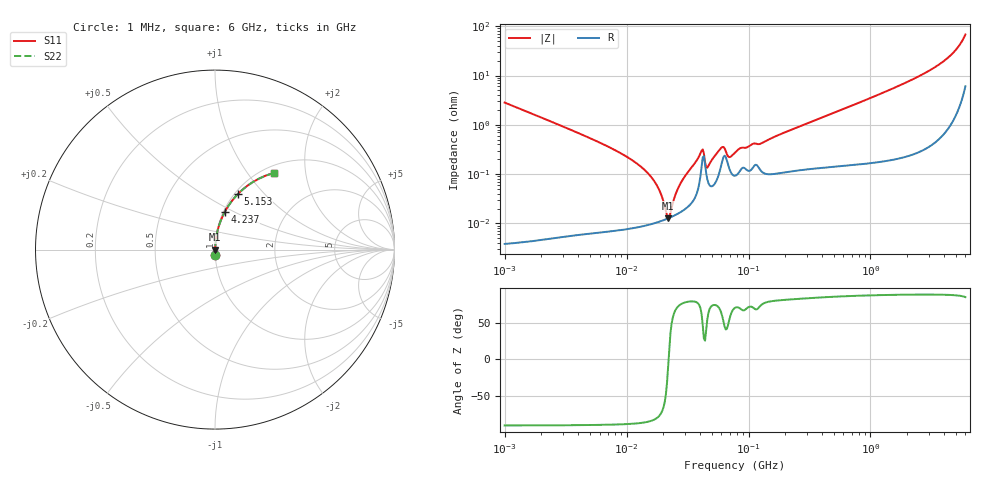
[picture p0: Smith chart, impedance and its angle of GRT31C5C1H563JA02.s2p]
!Murata Part Number: GRT31C5C1H563JA02
!These Parameters are Measured in Series Mode Connection
!Data Generated on Jun 19, 2026
!  o--ll--o
!Port1  Port2
!  o------o
!Operation Temp=25[degC], DC Bias Voltage=0[V]
!Freq. Start=1000[kHz] Stop=6[GHz] 401[Steps]
# Hz S RI R 50
!Freq.(Hz) S11(Real) S11(Imag) S21(Real) S21(Imag) S12(Real) S12(Imag) S22(Real) S22(Imag)
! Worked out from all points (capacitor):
!   401 points, 1 MHz to 6 GHz, reference 50 ohm
!   read as one part in series: C = 56.2 nF near 1.044 MHz
!   lowest |Z| = 12.8 mohm at 21.94 MHz (marker M1)
!   series resonance near 22.09 MHz, so ESL is about 920 pH
!   S11 on the Smith chart (normalised r, x): 1 MHz: 1.00, -0.06; 4.237 GHz: 1.02, +0.44; 5.153 GHz: 1.04, +0.72; 6 GHz: 1.12, +1.36
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1000000  0.000838 -0.0283  0.9992 0.0283  0.9992 0.0283  0.000838 -0.0283
4293785  9.96e-05 -0.00635  0.9999 0.00635  0.9999 0.00635  9.96e-05 -0.00635
1.16769e7  8.42e-05 -0.00176  0.9999 0.00176  0.9999 0.00176  8.42e-05 -0.00176
1.549236e7  9.56e-05 -0.000942  0.9999 0.000942  0.9999 0.000942  9.56e-05 -0.000942
1.843659e7  0.000108 -0.000476  0.9999 0.000476  0.9999 0.000476  0.000108 -0.000476
2.194036e7  0.000127 -1.83e-05  0.9999 1.83e-05  0.9999 1.83e-05  0.000127 -1.83e-05
2.291577e7  0.000133 9.76e-05  0.9999 -9.76e-05  0.9999 -9.76e-05  0.000133 9.76e-05
2.499862e7  0.000147 0.000334  0.9999 -0.000334  0.9999 -0.000334  0.000147 0.000334
2.727078e7  0.000166 0.000581  0.9998 -0.000581  0.9998 -0.000581  0.000166 0.000581
4.033799e7  0.000914 0.00247  0.9991 -0.00247  0.9991 -0.00247  0.000914 0.00247
4.213132e7  0.00218 0.00229  0.9978 -0.00229  0.9978 -0.00229  0.00218 0.00229
4.596069e7  0.000779 0.00111  0.9992 -0.00111  0.9992 -0.00111  0.000779 0.00111
5.966657e7  0.0015 0.00305  0.9985 -0.00305  0.9985 -0.00305  0.0015 0.00305
6.23192e7  0.00221 0.00277  0.9978 -0.00277  0.9978 -0.00277  0.00221 0.00277
6.947823e7  0.00131 0.00177  0.9987 -0.00177  0.9987 -0.00177  0.00131 0.00177
7.745967e7  0.000931 0.00258  0.9991 -0.00258  0.9991 -0.00258  0.000931 0.00258
3.325952e8  0.00141 0.0116  0.9986 -0.0116  0.9986 -0.0116  0.00141 0.0116
1.428092e9  0.00445 0.0505  0.9955 -0.0505  0.9955 -0.0505  0.00445 0.0505
2.802612e9  0.0156 0.1105  0.9844 -0.1105  0.9844 -0.1105  0.0156 0.1105
4.236675e9  0.0531 0.2074  0.9469 -0.2074  0.9469 -0.2074  0.0531 0.2074
5.152685e9  0.1274 0.3093  0.8726 -0.3093  0.8726 -0.3093  0.1274 0.3093
6e9  0.3304 0.4279  0.6696 -0.4279  0.6696 -0.4279  0.3304 0.4279
